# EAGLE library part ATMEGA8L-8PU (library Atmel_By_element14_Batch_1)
8-bit with 8KBytes In-System Programmable Flash
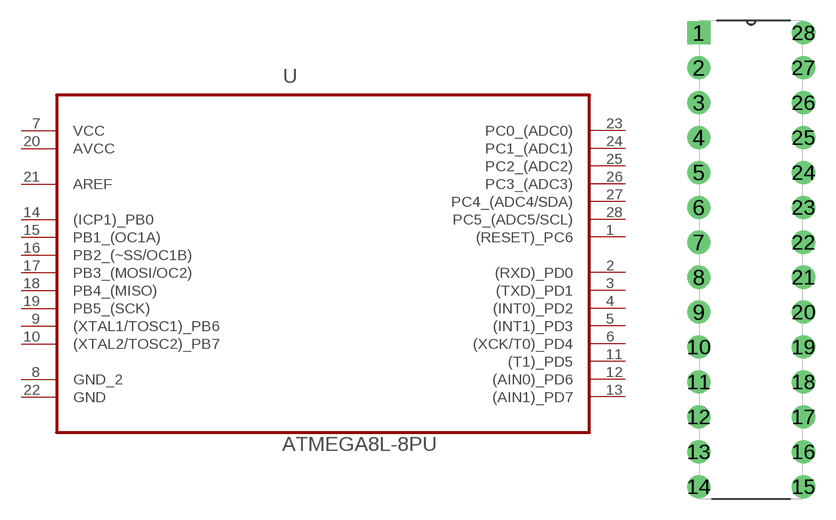
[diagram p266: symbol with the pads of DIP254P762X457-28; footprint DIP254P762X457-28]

Designator prefix U

## ATMEGA8L-8PU (DESCRIPTION: 8-bit with 8KBytes In-System Programmable Flash; MPN: ATMEGA8L-8PU; OC_FARNELL: 9171533; OC_NEWARK: 01M6903; PACKAGE: PCDIP-28; SUPPLIER: ATMEL)  [DIP254P762X457-28]
1  (RESET)_PC6
2  (RXD)_PD0
3  (TXD)_PD1
4  (INT0)_PD2
5  (INT1)_PD3
6  (XCK/T0)_PD4
7  VCC  pwr
8  GND_2  pas
9  (XTAL1/TOSC1)_PB6  in
10  (XTAL2/TOSC2)_PB7  in
11  (T1)_PD5
12  (AIN0)_PD6
13  (AIN1)_PD7
14  (ICP1)_PB0
15  PB1_(OC1A)
16  PB2_(~SS/OC1B)
17  PB3_(MOSI/OC2)
18  PB4_(MISO)
19  PB5_(SCK)
20  AVCC  pwr
21  AREF  in
22  GND  pas
23  PC0_(ADC0)
24  PC1_(ADC1)
25  PC2_(ADC2)
26  PC3_(ADC3)
27  PC4_(ADC4/SDA)
28  PC5_(ADC5/SCL)

## Footprint DIP254P762X457-28 (pad centres in mm)
drill 1.118 square: 1 -7.62,33.02
drill 1.118: 2 -7.62,30.48; 3 -7.62,27.94; 4 -7.62,25.4; 5 -7.62,22.86; 6 -7.62,20.32; 7 -7.62,17.78; 8 -7.62,15.24; 9 -7.62,12.7; 10 -7.62,10.16; 11 -7.62,7.62; 12 -7.62,5.08; 13 -7.62,2.54; 14 -7.62,0; 15 0,0; 16 0,2.54; 17 0,5.08; 18 0,7.62; 19 0,10.16; 20 0,12.7; 21 0,15.24; 22 0,17.78; 23 0,20.32; 24 0,22.86; 25 0,25.4; 26 0,27.94; 27 0,30.48; 28 0,33.02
